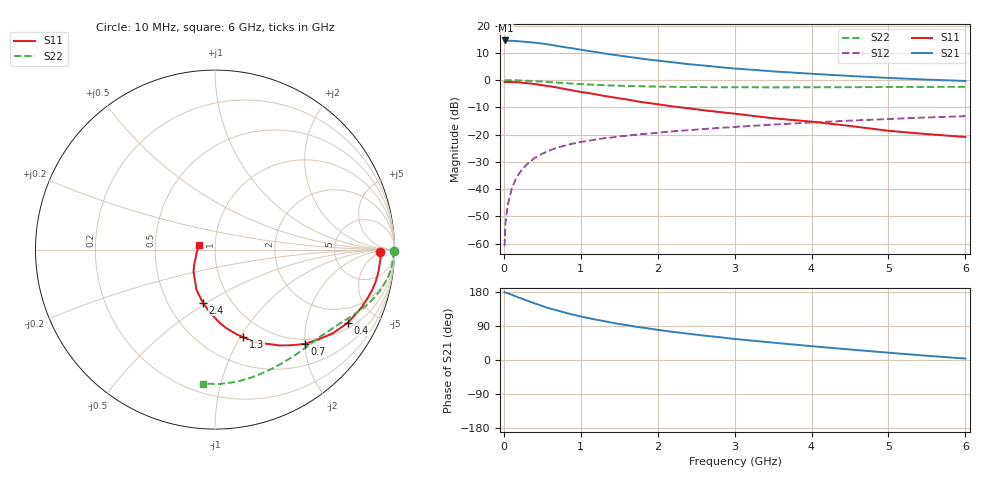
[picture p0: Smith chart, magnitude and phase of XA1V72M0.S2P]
! SIEMENS Discrete & RF Semiconductors
! BFY180
! Si NPN RF Bipolar Junction Transistor in MICRO-X
! VCE = 1.75 V  IC = 2 mA
! Common Emitter S-Parameters:  May  1997
# GHz  S  MA  R  50
!  f  S11  S21  S12  S22
! GHz  MAG  ANG  MAG  ANG  MAG  ANG  MAG  ANG
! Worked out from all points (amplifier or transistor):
!   36 points, 10 MHz to 6 GHz, reference 50 ohm
!   highest |S21| = 14.5 dB at 20 MHz (marker M1)
!   |S21| within 3 dB of that: start of sweep to 919.3 MHz
!   unconditionally stable (mu >= 1): 2.335 GHz to end of sweep
!   at 250 MHz: K = 0.15, MSG = 23.2 dB, |S12| = -32.3 dB
!   at 1.4 GHz: K = 0.76, MSG = 15.2 dB, |S12| = -21.1 dB
!   at 6 GHz: K = 1.10, MAG = 4.5 dB, |S12| = -13.2 dB
!   S11 on the Smith chart (normalised r, x): 10 MHz: 24, -4; 400 MHz: 1.23, -3.51; 700 MHz: 0.90, -2.00; 1.3 GHz: 0.78, -1.03; 2.4 GHz: 0.74, -0.48; 6 GHz: 0.84, +0.04
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0.01  0.922 -0.7  5.225 179.2  0.0009 81.1  0.9948 -0.3
0.02  0.9228 -1.7  5.321 178.3  0.0023 95.3  0.9963 -0.6
0.05  0.9228 -3.6  5.237 176.2  0.005 86.5  0.994 -1.7
0.1  0.9192 -7.4  5.249 172.3  0.0099 86.9  0.9905 -3.5
0.15  0.9132 -11.3  5.198 168.3  0.0147 83.3  0.9904 -5.2
0.3  0.8773 -21.7  4.998 156.7  0.0285 77.0  0.97 -10.1
0.4  0.8459 -28.7  4.848 149.4  0.0373 72.6  0.9545 -13.0
0.5  0.8062 -35.2  4.671 142.4  0.0446 68.7  0.934 -15.9
0.6  0.766 -40.6  4.447 135.7  0.0516 65.2  0.9147 -18.3
0.7  0.7262 -46.3  4.211 130.6  0.0579 62.2  0.896 -20.6
0.9  0.642 -56.3  3.805 119.6  0.0684 57.4  0.8591 -24.5
1.1  0.5779 -64.4  3.416 110.7  0.0769 53.4  0.8294 -27.9
1.3  0.513 -72.1  3.086 102.6  0.0856 50.7  0.8056 -31.0
1.5  0.4624 -78.8  2.812 95.0  0.0924 48.4  0.7876 -33.9
1.7  0.4155 -85.4  2.574 88.4  0.0989 46.7  0.7717 -36.6
2.2  0.3281 -98.2  2.112 74.2  0.115 42.7  0.7519 -43.4
2.4  0.3033 -102.8  1.956 69.3  0.1204 41.4  0.7455 -46.0
3  0.2421 -115.5  1.629 55.6  0.1381 37.2  0.7375 -53.8
3.5  0.1992 -124.4  1.443 45.8  0.1526 34.0  0.735 -60.3
4.5  0.144 -143.9  1.187 27.7  0.1802 26.9  0.7405 -73.7
5.5  0.1022 -172.7  1.02 11.2  0.2062 18.9  0.7494 -88.1
6  0.0903 164.4  0.962 3.8  0.218 14.7  0.7498 -95.3
